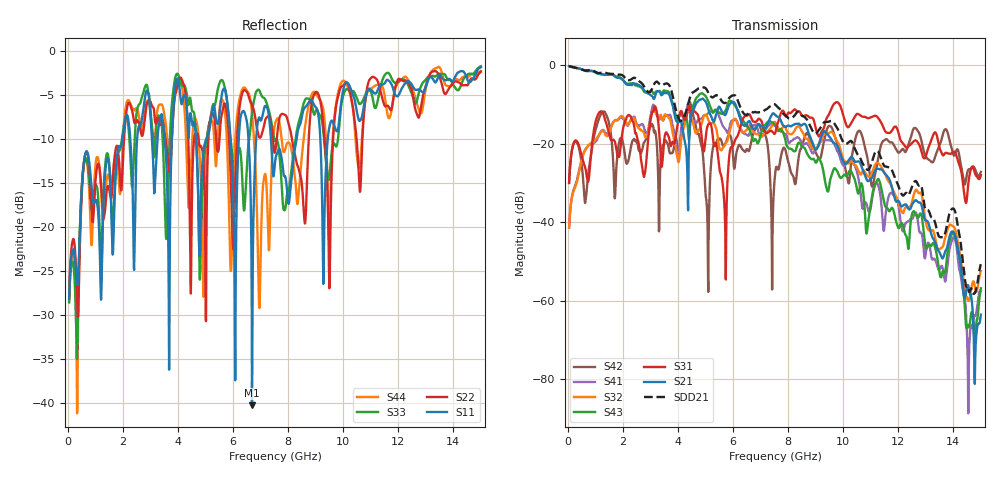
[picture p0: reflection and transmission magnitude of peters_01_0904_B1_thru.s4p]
# MHZ S RI R 50.00
! FREQ  S11  S12  S13  S14
!  S21  S22  S23  S24
!  S31  S32  S33  S34
!  S41  S42  S43  S44
!  REAL  IMAG  REAL  IMAG  REAL  IMAG  REAL  IMAG
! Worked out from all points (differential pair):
!   1496 points, 50 MHz to 15 GHz, reference 50 ohm
!   strongest paths, dB at 50 MHz, 3.79 GHz, 7.53 GHz, 11.27 GHz, 15 GHz:
!     S21: -0.2, -9.8, -12.6, -26.3, -63.6
!     S31: -30.0, -19.7, -17.3, -13.4, -28.0
!     S43: -0.2, -9.3, -15.1, -28.9, -56.8
!     S32: -41.3, -16.4, -14.5, -24.9, -52.4
!     S41: -41.3, -14.7, -15.5, -30.6, -57.5
!     S42: -30.0, -22.4, -27.6, -23.7, -27.2
!   taken as a pair (ports 1,3 in; 2,4 out), SDD21 dB: -0.2, -7.1, -10.0, -21.9, -50.7
!   lowest |S11| = -40.3 dB at 6.69 GHz (marker M1), VSWR 1.02, Z = 49.5 - j0.847 ohm
!   |S11| at or under -10 dB: start of sweep to 1.988 GHz; 4.661 GHz to 5.03 GHz (369.3 MHz wide, 7.62 % of centre); 7.378 GHz to 8.309 GHz (931.4 MHz wide, 11.9 % of centre)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
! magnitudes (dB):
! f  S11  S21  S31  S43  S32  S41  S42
! 50 MHz  -28.2  -0.2  -30.0  -0.2  -41.3  -41.3  -30.0
! 4.4 GHz  -9.4  -20.7  -9.7  -18.9  -11.3  -9.9  -9.7
! 5.07 GHz  -9.7  -10.3  -15.6  -8.7  -13.2  -12.4  -39.0
! 5.72 GHz  -4.5  -12.6  -42.7  -11.6  -20.1  -16.2  -20.0
! 6.69 GHz  -40.3  -15.8  -13.9  -18.3  -15.9  -15.4  -18.5
! 7.43 GHz  -13.0  -12.4  -16.9  -14.5  -15.2  -15.1  -46.7
! 15 GHz  -1.9  -63.6  -28.0  -56.8  -52.4  -57.5  -27.2
